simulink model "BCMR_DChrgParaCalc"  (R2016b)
settings: Solver=FixedStepDiscrete  StartTime=0.0  StopTime=10  FixedStep=0.01  RelTol=1e-3  EnableMultiTasking=on
undefined symbols (not defined in the file or in its folder): BCMR_ahDChgBattNominalCapa_C, BCMR_bCurrCalSelect_C, BCMR_bCurrIncDeltaLimEna_C, BCMR_bDChrgFulChkTenEna_C, BCMR_bDChrgFulChkThreeEna_C, BCMR_cntCoolDFC_CW, BCMR_cntSoh_CW, BCMR_G1E0PlatformSwPara_C, BCMR_iCurrDcr_C, BCMR_iDcChrgCurrAbnorm_T, BCMR_iDcChrgCurrAbnormMAP_T, BCMR_iDcChrgCurrNew_T, BCMR_iDcChrgCurrNewMAP_T, BCMR_iDcChrgCurrOld_T, BCMR_iDcChrgCurrOldAbnorm_T, BCMR_iDcChrgCurrOldAbnormMAP_T, BCMR_iDcChrgCurrOldMAP_T, BCMR_iDCCurrDecStep_C, BCMR_iDCCurrDecThrd_C, BCMR_iDCCurrDeltaLim_C, BCMR_iDCCurrDiff_C, BCMR_iDCCurrFil_C, BCMR_iDCCurrIncStep_C, BCMR_iDCCurrIncThrd_C, BCMR_iDChrgCurrCutOff_C, BCMR_kmAcmDist_C, BCMR_numCcsPwrSelc_C, BCMR_numCellVoltFull_C, BCMR_numCellVoltFullThree_C, BCMR_numCurrCalcEna, BCMR_pCcsPwrSelc_C, BCMR_pctBmsPwrRdc_C, BCMR_rCurrDcr_C, BCMR_rCurrIcr_C, BCMR_rDchrgLoadCoef_C, BCMR_tBattTempMaxFil_C, BCMR_tBattTempSelcLmtDwn_C, BCMR_tBattTempSelcLmtUp_C, BCMR_tDcChrgCellTemp1_A, BCMR_tDcChrgCellTemp2_A, BCMR_tDcChrgCellTemp_A, BCMR_tDchrgLoadLmt_C, BCMR_tiBattTempMaxFilDly_C, BCMR_tiBattTempSwitch_C, BCMR_tiCellVoltFullCnt_C, BCMR_tiCellVoltMaxFilDly_C, BCMR_tiCurrHysTimeDelay_C, BCMR_tiDcChrgPwrCCSDebs_C, BCMR_tiDChgFullPreHold_C, BCMR_tiDChrgCurrReqCalDly_C, BCMR_tiDChrgDetParaDebs_C, BCMR_tiDChrgFullBase_C, BCMR_tiDChrgFullDebs_C, BCMR_tiDChrgFulParaDebs_C, BCMR_tiDChrgFulWait_C, BCMR_tiDChrgParaBase_C, BCMR_tiHoldOnToCurrCalcOff_C, BCMR_tTempDisMapX_A, BCMR_tTempDisMapY_A, BCMR_uBattVoltOff_C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
libraries: simulink x34
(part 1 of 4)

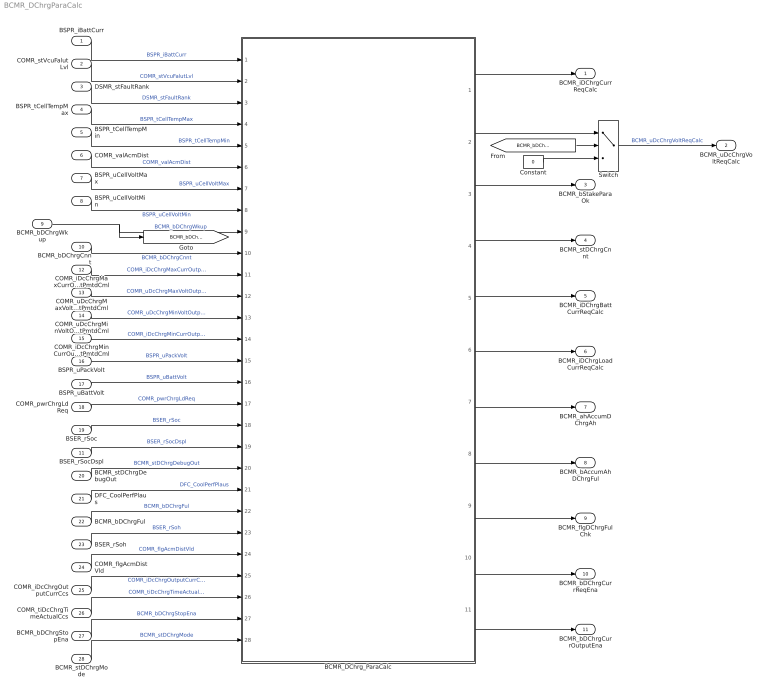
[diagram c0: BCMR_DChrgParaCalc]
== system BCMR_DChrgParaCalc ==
  BSPR_iBattCurr : Inport
  COMR_stVcuFalutLvl : Inport  Port=2
  DSMR_stFaultRank : Inport  Port=3
  BSPR_tCellTempMax : Inport  Port=4
  BSPR_tCellTempMin : Inport  Port=5
  COMR_valAcmDist : Inport  Port=6
  BSPR_uCellVoltMax : Inport  Port=7
  BSPR_uCellVoltMin : Inport  Port=8
  BCMR_bDChrgWkup : Inport  Port=9
  BCMR_bDChrgCnnt : Inport  Port=10
  BSER_rSocDspl : Inport  Port=11
  COMR_iDcChrgMaxCurrOutputPmtdCml : Inport  Port=12
  COMR_uDcChrgMaxVoltOutputPmtdCml : Inport  Port=13
  COMR_uDcChrgMinVoltOutputPmtdCml : Inport  Port=14
  COMR_iDcChrgMinCurrOutputPmtdCml : Inport  Port=15
  BSPR_uPackVolt : Inport  Port=16
  BSPR_uBattVolt : Inport  Port=17
  COMR_pwrChrgLdReq : Inport  Port=18
  BSER_rSoc : Inport  Port=19
  BCMR_stDChrgDebugOut : Inport  Port=20
  DFC_CoolPerfPlaus : Inport  Port=21
  BCMR_bDChrgFul : Inport  Port=22
  BSER_rSoh : Inport  Port=23
  COMR_flgAcmDistVld : Inport  Port=24
  COMR_iDcChrgOutputCurrCcs : Inport  Port=25
  COMR_tiDcChrgTimeActualCcs : Inport  Port=26
  BCMR_bDChrgStopEna : Inport  Port=27
  BCMR_stDChrgMode : Inport  Port=28
  BCMR_DChrg_ParaCalc : Subsystem
  Constant : Constant  Value=0
  Switch : Switch  Criteria=u2 > Threshold  OutDataTypeStr=single
  BCMR_iDChrgCurrReqCalc : Outport
  BCMR_uDcChrgVoltReqCalc : Outport  Port=2
  BCMR_bStakeParaOk : Outport  Port=3
  BCMR_stDChrgCnnt : Outport  Port=4
  BCMR_iDChrgBattCurrReqCalc : Outport  Port=5
  BCMR_iDChrgLoadCurrReqCalc : Outport  Port=6
  BCMR_ahAccumDChrgAh : Outport  Port=7  InitialOutput=[0]
  BCMR_bAccumAhDChrgFul : Outport  Port=8  InitialOutput=[0]
  BCMR_flgDChrgFulChk : Outport  Port=9
  BCMR_bDChrgCurrReqEna : Outport  Port=10  OutputWhenDisabled=reset  InitialOutput=[0]
  BCMR_bDChrgCurrOutputEna : Outport  Port=11  OutputWhenDisabled=reset  InitialOutput=[0]
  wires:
  BSPR_iBattCurr/1 -> BCMR_DChrg_ParaCalc/1(BSPR_iBattCurr)  "BSPR_iBattCurr"
  COMR_stVcuFalutLvl/1 -> BCMR_DChrg_ParaCalc/2(COMR_stVcuFalutLvl)  "COMR_stVcuFalutLvl"
  DSMR_stFaultRank/1 -> BCMR_DChrg_ParaCalc/3(DSMR_stFaultRank)  "DSMR_stFaultRank"
  BSPR_tCellTempMax/1 -> BCMR_DChrg_ParaCalc/4(BSPR_tBattTempMax)  "BSPR_tCellTempMax"
  BSPR_tCellTempMin/1 -> BCMR_DChrg_ParaCalc/5(BSPR_tBattTempMin)  "BSPR_tCellTempMin"
  COMR_valAcmDist/1 -> BCMR_DChrg_ParaCalc/6(COMR_valAcmDist)  "COMR_valAcmDist"
  BSPR_uCellVoltMax/1 -> BCMR_DChrg_ParaCalc/7(BSPR_uCellVoltMax)  "BSPR_uCellVoltMax"
  BSPR_uCellVoltMin/1 -> BCMR_DChrg_ParaCalc/8(BSPR_uCellVoltMin)  "BSPR_uCellVoltMin"
  BCMR_bDChrgWkup/1 -> [BCMR_bDChrgWkup], BCMR_DChrg_ParaCalc/9(BCMR_bDChrgWkup)  "BCMR_bDChrgWkup"
  BCMR_bDChrgCnnt/1 -> BCMR_DChrg_ParaCalc/10(BCMR_bDChrgCnnt)  "BCMR_bDChrgCnnt"
  BSER_rSocDspl/1 -> BCMR_DChrg_ParaCalc/19(BSER_rSocDspl)  "BSER_rSocDspl"
  COMR_iDcChrgMaxCurrOutputPmtdCml/1 -> BCMR_DChrg_ParaCalc/11(COMR_iDcChrgMaxCurrOutputPmtdCml)  "COMR_iDcChrgMaxCurrOutputPmtdCml"
  COMR_uDcChrgMaxVoltOutputPmtdCml/1 -> BCMR_DChrg_ParaCalc/12(COMR_uDcChrgMaxVoltOutputPmtdCml)  "COMR_uDcChrgMaxVoltOutputPmtdCml"
  COMR_uDcChrgMinVoltOutputPmtdCml/1 -> BCMR_DChrg_ParaCalc/13(COMR_uDcChrgMinVoltOutputPmtdCml)  "COMR_uDcChrgMinVoltOutputPmtdCml"
  COMR_iDcChrgMinCurrOutputPmtdCml/1 -> BCMR_DChrg_ParaCalc/14(COMR_iDcChrgMinCurrOutputPmtdCml)  "COMR_iDcChrgMinCurrOutputPmtdCml"
  BSPR_uPackVolt/1 -> BCMR_DChrg_ParaCalc/15(BSPR_uPackVolt)  "BSPR_uPackVolt"
  BSPR_uBattVolt/1 -> BCMR_DChrg_ParaCalc/16(BSPR_uBattVolt)  "BSPR_uBattVolt"
  BCMR_DChrg_ParaCalc/1(BCMR_iDChrgCurrReqCalc) -> BCMR_iDChrgCurrReqCalc/1
  BCMR_DChrg_ParaCalc/3(BCMR_bStakeParaOk) -> BCMR_bStakeParaOk/1
  BCMR_DChrg_ParaCalc/4("BCMR_stDChrgCnnt ") -> BCMR_stDChrgCnnt/1
  COMR_pwrChrgLdReq/1 -> BCMR_DChrg_ParaCalc/17(COMR_pwrChrgLdReq)  "COMR_pwrChrgLdReq"
  BCMR_DChrg_ParaCalc/5(BCMR_iDChrgBattCurrReqCalc) -> BCMR_iDChrgBattCurrReqCalc/1
  BCMR_DChrg_ParaCalc/6(BCMR_iDChrgLoadCurrReqCalc) -> BCMR_iDChrgLoadCurrReqCalc/1
  BSER_rSoc/1 -> BCMR_DChrg_ParaCalc/18(BSER_rSoc)  "BSER_rSoc"
  BCMR_DChrg_ParaCalc/7(BCMR_ahAccumDChrgAh) -> BCMR_ahAccumDChrgAh/1
  BCMR_DChrg_ParaCalc/8(BCMR_bAccumAhDChrgFul) -> BCMR_bAccumAhDChrgFul/1
  BCMR_DChrg_ParaCalc/9(BCMR_flgDChrgFulChk) -> BCMR_flgDChrgFulChk/1
  BCMR_stDChrgDebugOut/1 -> BCMR_DChrg_ParaCalc/20(BCMR_stDChrgDebugOut)  "BCMR_stDChrgDebugOut"
  DFC_CoolPerfPlaus/1 -> BCMR_DChrg_ParaCalc/21(DFC_CoolPerfPlaus)  "DFC_CoolPerfPlaus"
  BCMR_bDChrgFul/1 -> BCMR_DChrg_ParaCalc/22(BCMR_bDChrgFul)  "BCMR_bDChrgFul"
  BSER_rSoh/1 -> BCMR_DChrg_ParaCalc/23(BSER_rSoh)  "BSER_rSoh"
  BCMR_DChrg_ParaCalc/10(BCMR_bDChrgCurrReqEna) -> BCMR_bDChrgCurrReqEna/1
  BCMR_DChrg_ParaCalc/11(BCMR_bDChrgCurrOutputEna) -> BCMR_bDChrgCurrOutputEna/1
  COMR_flgAcmDistVld/1 -> BCMR_DChrg_ParaCalc/24(COMR_flgAcmDistVld)  "COMR_flgAcmDistVld"
  COMR_iDcChrgOutputCurrCcs/1 -> BCMR_DChrg_ParaCalc/25(COMR_iDcChrgOutputCurrCcs)  "COMR_iDcChrgOutputCurrCcs"
  COMR_tiDcChrgTimeActualCcs/1 -> BCMR_DChrg_ParaCalc/26(COMR_tiDcChrgTimeActualCcs)  "COMR_tiDcChrgTimeActualCcs"
  BCMR_bDChrgStopEna/1 -> BCMR_DChrg_ParaCalc/27(BCMR_bDChrgStopEna)  "BCMR_bDChrgStopEna"
  BCMR_stDChrgMode/1 -> BCMR_DChrg_ParaCalc/28(BCMR_stDChrgMode)  "BCMR_stDChrgMode"
  Switch/1 -> BCMR_uDcChrgVoltReqCalc/1  "BCMR_uDcChrgVoltReqCalc"
  [BCMR_bDChrgWkup] -> Switch/2
  Constant/1 -> Switch/3
  BCMR_DChrg_ParaCalc/2(BCMR_uDcChrgVoltReqCalc) -> Switch/1

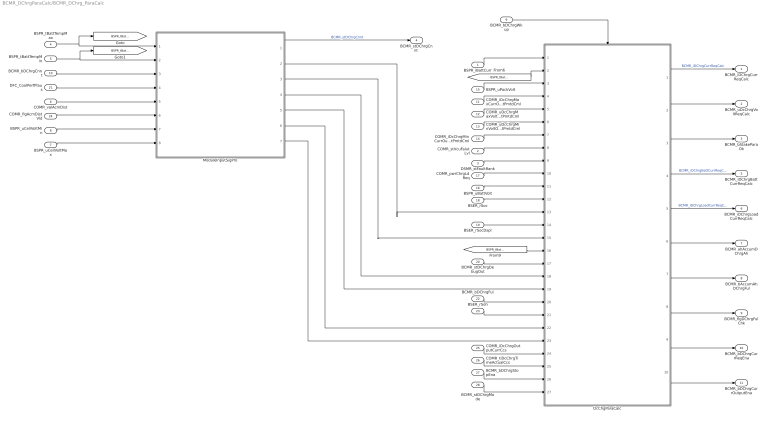
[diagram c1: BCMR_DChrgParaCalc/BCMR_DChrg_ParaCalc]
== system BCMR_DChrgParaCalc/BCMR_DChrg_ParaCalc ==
  BSPR_iBattCurr : Inport
  COMR_stVcuFalutLvl : Inport  Port=2
  DSMR_stFaultRank : Inport  Port=3
  BSPR_tBattTempMax : Inport  Port=4
  BSPR_tBattTempMin : Inport  Port=5
  COMR_valAcmDist : Inport  Port=6
  BSPR_uCellVoltMax : Inport  Port=7
  BSPR_uCellVoltMin : Inport  Port=8
  BCMR_bDChrgWkup : Inport  Port=9
  BCMR_bDChrgCnnt : Inport  Port=10
  COMR_iDcChrgMaxCurrOutputPmtdCml : Inport  Port=11
  COMR_uDcChrgMaxVoltOutputPmtdCml : Inport  Port=12
  COMR_uDcChrgMinVoltOutputPmtdCml : Inport  Port=13
  COMR_iDcChrgMinCurrOutputPmtdCml : Inport  Port=14
  BSPR_uPackVolt : Inport  Port=15
  BSPR_uBattVolt : Inport  Port=16
  COMR_pwrChrgLdReq : Inport  Port=17
  BSER_rSoc : Inport  Port=18
  BSER_rSocDspl : Inport  Port=19
  BCMR_stDChrgDebugOut : Inport  Port=20
  DFC_CoolPerfPlaus : Inport  Port=21
  BCMR_bDChrgFul : Inport  Port=22
  BSER_rSoh : Inport  Port=23
  COMR_flgAcmDistVld : Inport  Port=24
  COMR_iDcChrgOutputCurrCcs : Inport  Port=25
  COMR_tiDcChrgTimeActualCcs : Inport  Port=26
  BCMR_bDChrgStopEna : Inport  Port=27
  BCMR_stDChrgMode : Inport  Port=28
  DcChgParaCalc : Subsystem  TreatAsAtomicUnit=on
  ModuleInputSigPro : Subsystem  TreatAsAtomicUnit=on
  BCMR_iDChrgCurrReqCalc : Outport
  BCMR_uDcChrgVoltReqCalc : Outport  Port=2
  BCMR_bStakeParaOk : Outport  Port=3
  "BCMR_stDChrgCnnt " : Outport  Port=4
  BCMR_iDChrgBattCurrReqCalc : Outport  Port=5
  BCMR_iDChrgLoadCurrReqCalc : Outport  Port=6
  BCMR_ahAccumDChrgAh : Outport  Port=7  InitialOutput=[0]
  BCMR_bAccumAhDChrgFul : Outport  Port=8  InitialOutput=[0]
  BCMR_flgDChrgFulChk : Outport  Port=9
  BCMR_bDChrgCurrReqEna : Outport  Port=10  OutputWhenDisabled=reset  InitialOutput=[0]
  BCMR_bDChrgCurrOutputEna : Outport  Port=11  OutputWhenDisabled=reset  InitialOutput=[0]
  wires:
  BCMR_bDChrgWkup/1 -> DcChgParaCalc/Enable
  ModuleInputSigPro/1(BCMR_stDChrgCnnt) -> "BCMR_stDChrgCnnt "/1  "BCMR_stDChrgCnnt"
  BSPR_iBattCurr/1 -> DcChgParaCalc/1(BSPR_iBattCurr)
  BSPR_uBattVolt/1 -> DcChgParaCalc/11(BSPR_uBattVolt)
  BSPR_uPackVolt/1 -> DcChgParaCalc/3(BSPR_uPackVolt)
  COMR_iDcChrgMaxCurrOutputPmtdCml/1 -> DcChgParaCalc/4(COMR_iDcChrgMaxCurrOutputPmtdCml)
  COMR_uDcChrgMaxVoltOutputPmtdCml/1 -> DcChgParaCalc/5(COMR_uDcChrgMaxVoltOutputPmtdCml)
  COMR_uDcChrgMinVoltOutputPmtdCml/1 -> DcChgParaCalc/6(COMR_uDcChrgMinVoltOutputPmtdCml)
  COMR_iDcChrgMinCurrOutputPmtdCml/1 -> DcChgParaCalc/7(COMR_iDcChrgMinCurrOutputPmtdCml)
  COMR_stVcuFalutLvl/1 -> DcChgParaCalc/8(COMR_stVcuFalutLvl)
  DSMR_stFaultRank/1 -> DcChgParaCalc/9(DSMR_stFaultRank)
  DcChgParaCalc/2(BCMR_uDcChrgVoltReqCalc) -> BCMR_uDcChrgVoltReqCalc/1
  DcChgParaCalc/1(BCMR_iDChrgCurrReqCalc) -> BCMR_iDChrgCurrReqCalc/1  "BCMR_iDChrgCurrReqCalc"
  DcChgParaCalc/3(BCMR_bStakeParaOk) -> BCMR_bStakeParaOk/1
  COMR_pwrChrgLdReq/1 -> DcChgParaCalc/10(COMR_pwrChrgLdReq)
  DcChgParaCalc/4(BCMR_iDChrgBattCurrReqCalc) -> BCMR_iDChrgBattCurrReqCalc/1  "BCMR_iDChrgBattCurrReqCalc"
  DcChgParaCalc/5(BCMR_iDChrgLoadCurrReqCalc) -> BCMR_iDChrgLoadCurrReqCalc/1  "BCMR_iDChrgLoadCurrReqCalc"
  BSER_rSoc/1 -> DcChgParaCalc/12(BSER_rSoc)
  DcChgParaCalc/6(BCMR_ahAccumDChrgAh) -> BCMR_ahAccumDChrgAh/1
  DcChgParaCalc/7(BCMR_bAccumAhDChrgFul) -> BCMR_bAccumAhDChrgFul/1
  DcChgParaCalc/8(BCMR_flgDChrgFulChk) -> BCMR_flgDChrgFulChk/1
  BSER_rSocDspl/1 -> DcChgParaCalc/14(BSER_rSocDspl)
  BSPR_tBattTempMax/1 -> [BSPR_tBattTempMax], ModuleInputSigPro/1(BSPR_tBattTempMax)
  BSPR_tBattTempMin/1 -> ModuleInputSigPro/2(BSPR_tBattTempMin), [BSPR_tBattTempMin]
  [BSPR_tBattTempMin] -> DcChgParaCalc/2(BSPR_tBattTempMin)
  BSPR_uCellVoltMax/1 -> ModuleInputSigPro/8(BSPR_uCellVoltMin)
  [BSPR_tBattTempMax] -> DcChgParaCalc/16(BSPR_tBattTempMax)
  BSPR_uCellVoltMin/1 -> ModuleInputSigPro/7(BSPR_uCellVoltMax)
  BCMR_stDChrgDebugOut/1 -> DcChgParaCalc/17(BCMR_stDChrgDebugOut)
  ModuleInputSigPro/4(BCMR_uDcChrgCellVolt_A) -> DcChgParaCalc/18(BCMR_uDcChrgCellVolt_A)
  DFC_CoolPerfPlaus/1 -> ModuleInputSigPro/4(DFC_CoolPerfPlaus)
  ModuleInputSigPro/5(BCMR_bDChrgCoolAbnorm) -> DcChgParaCalc/19(BCMR_bDChrgCoolAbnorm)
  BCMR_bDChrgFul/1 -> DcChgParaCalc/20(BCMR_bDChrgFul)
  BSER_rSoh/1 -> DcChgParaCalc/21(BSER_rSoh)
  DcChgParaCalc/9(BCMR_bDChrgCurrReqEna) -> BCMR_bDChrgCurrReqEna/1
  DcChgParaCalc/10(BCMR_bDChrgCurrOutputEna) -> BCMR_bDChrgCurrOutputEna/1
  BCMR_bDChrgCnnt/1 -> ModuleInputSigPro/3(BCMR_bDChrgCnnt)
  COMR_valAcmDist/1 -> ModuleInputSigPro/5(COMR_valAcmDist)
  COMR_flgAcmDistVld/1 -> ModuleInputSigPro/6(COMR_flgAcmDistVld)
  ModuleInputSigPro/6(BCMR_tDcChrgCellTemp_A) -> DcChgParaCalc/22(BCMR_tDcChrgCellTemp_A)
  ModuleInputSigPro/7(BCMR_bDChrgDistLmt) -> DcChgParaCalc/23(BCMR_bDChrgDistLmt)
  COMR_tiDcChrgTimeActualCcs/1 -> DcChgParaCalc/25(COMR_tiDcChrgTimeActualCcs)
  COMR_iDcChrgOutputCurrCcs/1 -> DcChgParaCalc/24(COMR_iDcChrgOutputCurrCcs)
  BCMR_bDChrgStopEna/1 -> DcChgParaCalc/26(BCMR_bDChrgStopEna)
  BCMR_stDChrgMode/1 -> DcChgParaCalc/27(BCMR_stDChrgMode)
  ModuleInputSigPro/2(BCMR_uCellVoltMax) -> DcChgParaCalc/13(BSPR_uCellVoltMax)
  ModuleInputSigPro/3(BCMR_uCellVoltMin) -> DcChgParaCalc/15(BSPR_uCellVoltMin)

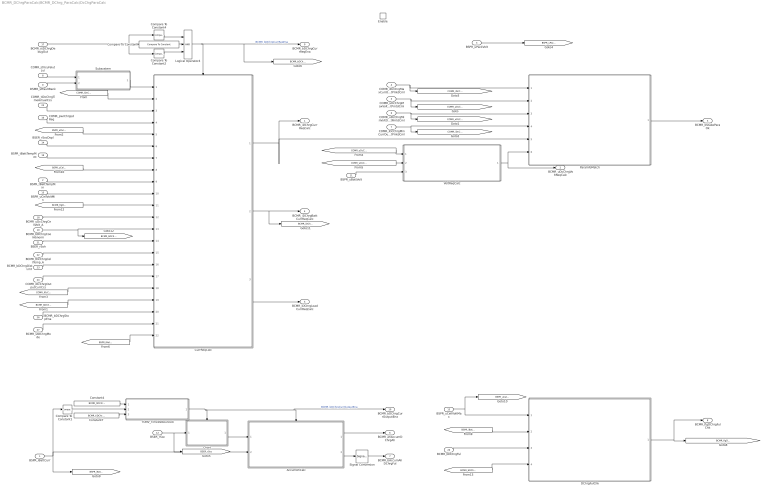
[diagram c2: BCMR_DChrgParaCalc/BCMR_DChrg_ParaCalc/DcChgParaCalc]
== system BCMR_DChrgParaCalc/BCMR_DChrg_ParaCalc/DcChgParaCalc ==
  BSPR_iBattCurr : Inport
  BSPR_tBattTempMin : Inport  Port=2
  BSPR_uPackVolt : Inport  Port=3
  COMR_iDcChrgMaxCurrOutputPmtdCml : Inport  Port=4
  COMR_uDcChrgMaxVoltOutputPmtdCml : Inport  Port=5
  COMR_uDcChrgMinVoltOutputPmtdCml : Inport  Port=6
  COMR_iDcChrgMinCurrOutputPmtdCml : Inport  Port=7
  COMR_stVcuFalutLvl : Inport  Port=8
  DSMR_stFaultRank : Inport  Port=9
  COMR_pwrChrgLdReq : Inport  Port=10
  BSPR_uBattVolt : Inport  Port=11
  BSER_rSoc : Inport  Port=12
  BSPR_uCellVoltMax : Inport  Port=13
  BSER_rSocDspl : Inport  Port=14
  BSPR_uCellVoltMin : Inport  Port=15
  BSPR_tBattTempMax : Inport  Port=16
  BCMR_stDChrgDebugOut : Inport  Port=17
  BCMR_uDcChrgCellVolt_A : Inport  Port=18
  BCMR_bDChrgCoolAbnorm : Inport  Port=19
  BCMR_bDChrgFul : Inport  Port=20
  BSER_rSoh : Inport  Port=21
  BCMR_tDcChrgCellTemp_A : Inport  Port=22
  BCMR_bDChrgDistLmt : Inport  Port=23
  COMR_iDcChrgOutputCurrCcs : Inport  Port=24
  COMR_tiDcChrgTimeActualCcs : Inport  Port=25
  BCMR_bDChrgStopEna : Inport  Port=26
  BCMR_stDChrgMode : Inport  Port=27
  Enable : EnablePort  StatesWhenEnabling=reset
  AccumAhCalc : Subsystem  TreatAsAtomicUnit=on
  Chart : Stateflow chart  TreatAsAtomicUnit=on
  Compare To Constant : simulink/Logic and Bit Operations/Compare To Constant  relop=>=  const=BCMR_numCurrCalcEna  OutDataTypeStr=boolean
  Compare To Constant1 : simulink/Logic and Bit Operations/Compare To Constant  relop=<=  const=-5  OutDataTypeStr=boolean
  Compare To Constant2 : simulink/Logic and Bit Operations/Compare To Constant  relop=<  const=34  OutDataTypeStr=boolean
  Compare To Constant4 : simulink/Logic and Bit Operations/Compare To Constant  relop=~=  const=24  OutDataTypeStr=boolean
  Constant4 : Constant  Value=BCMR_tiDChrgDetParaDebs_C
  Constant7 : Constant  Value=BCMR_tiDChrgParaBase_C
  CurrReqCalc : Subsystem  TreatAsAtomicUnit=on
  DChrgFulChk : Subsystem  TreatAsAtomicUnit=on
  Logical Operator4 : Logic  Inputs=3  AllPortsSameDT=off  OutDataTypeStr=boolean
  ParaInfoMatch : Subsystem
  Signal Conversion : SignalConversion  OverrideOpt=off
  Subsystem : Subsystem
  TONV_TimeDebounce4 : Subsystem  TreatAsAtomicUnit=on
  VoltReqCalc : Subsystem  TreatAsAtomicUnit=on
  BCMR_iDChrgCurrReqCalc : Outport  OutputWhenDisabled=reset  InitialOutput=[0]
  BCMR_uDcChrgVoltReqCalc : Outport  Port=2  InitialOutput=[0]
  BCMR_bStakeParaOk : Outport  Port=3  OutputWhenDisabled=reset  InitialOutput=[0]
  BCMR_iDChrgBattCurrReqCalc : Outport  Port=4  OutputWhenDisabled=reset  InitialOutput=[0]
  BCMR_iDChrgLoadCurrReqCalc : Outport  Port=5  OutputWhenDisabled=reset  InitialOutput=[0]
  BCMR_ahAccumDChrgAh : Outport  Port=6  OutputWhenDisabled=reset  InitialOutput=[0]
  BCMR_bAccumAhDChrgFul : Outport  Port=7  InitialOutput=[0]
  BCMR_flgDChrgFulChk : Outport  Port=8  OutputWhenDisabled=reset  InitialOutput=[0]
  BCMR_bDChrgCurrReqEna : Outport  Port=9  OutputWhenDisabled=reset  InitialOutput=[0]
  BCMR_bDChrgCurrOutputEna : Outport  Port=10  OutputWhenDisabled=reset  InitialOutput=[0]
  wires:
  VoltReqCalc/1(BCMR_uDcChrgVoltReqCalc) -> ParaInfoMatch/6(BCMR_uDcChrgVoltReqCalc), BCMR_uDcChrgVoltReqCalc/1
  ParaInfoMatch/1(BCMR_bStakeParaOk) -> BCMR_bStakeParaOk/1
  COMR_uDcChrgMaxVoltOutputPmtdCml/1 -> [COMR_uDcChrgMaxVoltOutputPmtdCml], ParaInfoMatch/2(COMR_uDcChrgMaxVoltOutputPmtdCml)
  COMR_uDcChrgMinVoltOutputPmtdCml/1 -> [COMR_uDcChrgMinVoltOutputPmtdCml], ParaInfoMatch/3(COMR_uDcChrgMinVoltOutputPmtdCml)
  [COMR_uDcChrgMaxVoltOutputPmtdCml] -> VoltReqCalc/1(COMR_uDcChrgMaxVoltOutputPmtdCml)
  [COMR_uDcChrgMinVoltOutputPmtdCml] -> VoltReqCalc/2(COMR_uDcChrgMinVoltOutputPmtdCml)
  COMR_iDcChrgMaxCurrOutputPmtdCml/1 -> ParaInfoMatch/1(COMR_iDcChrgMaxCurrOutputPmtdCml), [COMR_iDcChrgMaxCurrOutputPmtdCml]
  COMR_iDcChrgMinCurrOutputPmtdCml/1 -> [COMR_iDcChrgMinCurrOutputPmtdCml], ParaInfoMatch/4(COMR_iDcChrgMinCurrOutputPmtdCml)
  BSPR_uPackVolt/1 -> [BSPR_uPackVolt]
  BSPR_iBattCurr/1 -> AccumAhCalc/2(BSPR_iBattCurr), [BSPR_iBattCurr], Compare To Constant1/1
  [COMR_iDcChrgMaxCurrOutputPmtdCml] -> CurrReqCalc/2(COMR_iDcChrgMaxCurrOutputPmtdCml)
  COMR_stVcuFalutLvl/1 -> Subsystem/1(COMR_stVcuFalutLvl)
  DSMR_stFaultRank/1 -> Subsystem/2(DSMR_stFaultRank)
  Subsystem/1(BCMR_flgDChrgPwrRdc) -> CurrReqCalc/1(BCMR_flgDChrgPwrRdc)
  [BSPR_uPackVolt] -> CurrReqCalc/5(BSPR_uPackVolt)
  COMR_pwrChrgLdReq/1 -> CurrReqCalc/4(COMR_pwrChrgLdReq)
  CurrReqCalc/3(BCMR_iDChrgLoadCurrReqCalc) -> BCMR_iDChrgLoadCurrReqCalc/1
  CurrReqCalc/2(BCMR_iDChrgBattCurrReqCalc) -> BCMR_iDChrgBattCurrReqCalc/1, [BCMR_iDChrgBattCurrReqCalc]
  BSER_rSoc/1 -> [BSER_rSoc], Chart/1(BSER_rSoc)
  Chart/1(BCMR_rSocInit) -> AccumAhCalc/1(BCMR_rSocInit)
  AccumAhCalc/1(BCMR_ahAccumDChrgAh) -> BCMR_ahAccumDChrgAh/1
  AccumAhCalc/2(BCMR_bAccumAhDChrgFul) -> Signal Conversion/1
  BSER_rSocDspl/1 -> CurrReqCalc/6(BSER_rSocDspl)
  Compare To Constant1/1 -> TONV_TimeDebounce4/2(u)
  TONV_TimeDebounce4/1(y) -> BCMR_bDChrgCurrOutputEna/1, AccumAhCalc/Enable, Chart/Trigger  "BCMR_bDChrgCurrOutputEna"
  Constant7/1 -> TONV_TimeDebounce4/3(dT)
  Constant4/1 -> TONV_TimeDebounce4/1(T)
  BSPR_tBattTempMin/1 -> CurrReqCalc/9(BSPR_tBattTempMin)
  BSPR_uCellVoltMin/1 -> CurrReqCalc/10(BSPR_uCellVoltMin)
  [BSPR_uCellVoltMax] -> CurrReqCalc/8(BSPR_uCellVoltMax)
  BSPR_tBattTempMax/1 -> CurrReqCalc/7(BSPR_tBattTempMax)
  [BCMR_flgDChrgFulChk] -> CurrReqCalc/11(BCMR_flgDChrgFulChk)
  DChrgFulChk/1(BCMR_flgDChrgFulChk) -> BCMR_flgDChrgFulChk/1, [BCMR_flgDChrgFulChk]
  BCMR_stDChrgDebugOut/1 -> Compare To Constant4/1, Compare To Constant/1, Compare To Constant2/1
  COMR_tiDcChrgTimeActualCcs/1 -> CurrReqCalc/3(COMR_tiDcChrgTimeActualCcs)
  BCMR_uDcChrgCellVolt_A/1 -> CurrReqCalc/12(BCMR_uDcChrgCellVolt_A)
  [BSPR_iBattCurr] -> DChrgFulChk/2(BSPR_iBattCurr)
  BSPR_uCellVoltMax/1 -> DChrgFulChk/1(BSPR_uCellVoltMax), [BSPR_uCellVoltMax]
  BCMR_bDChrgFul/1 -> DChrgFulChk/3(BCMR_bDChrgFul)
  BSER_rSoh/1 -> CurrReqCalc/14(BSER_rSoh)
  [BCMR_bDChrgCoolAbnorm] -> DChrgFulChk/4(BCMR_bDChrgCoolAbnorm)
  Logical Operator4/1 -> [BCMR_bDChrgCurrReqEna], BCMR_bDChrgCurrReqEna/1, CurrReqCalc/Enable  "BCMR_bDChrgCurrReqEna"
  Compare To Constant4/1 -> Logical Operator4/1
  Compare To Constant/1 -> Logical Operator4/2
  Compare To Constant2/1 -> Logical Operator4/3
  BCMR_bDChrgCoolAbnorm/1 -> [BCMR_bDChrgCoolAbnorm], CurrReqCalc/13(BCMR_bDChrgCoolAbnorm)
  CurrReqCalc/1(BCMR_iDChrgCurrReqCalc) -> ParaInfoMatch/5(BCMR_iDChrgCurrReqCalc), BCMR_iDChrgCurrReqCalc/1
  BCMR_tDcChrgCellTemp_A/1 -> CurrReqCalc/15(BCMR_tDcChrgCellTemp_A)
  BCMR_bDChrgDistLmt/1 -> CurrReqCalc/16(BCMR_bDChrgDistLmt)
  BSPR_uBattVolt/1 -> VoltReqCalc/3(BSPR_uBattVolt)
  [COMR_iDcChrgMinCurrOutputPmtdCml] -> CurrReqCalc/18(COMR_iDcChrgMinCurrOutputPmtdCml)
  COMR_iDcChrgOutputCurrCcs/1 -> CurrReqCalc/17(COMR_iDcChrgOutputCurrCcs)
  [BCMR_bDChrgCurrReqEna] -> CurrReqCalc/19(BCMR_bDChrgCurrReqEna)
  BCMR_bDChrgStopEna/1 -> CurrReqCalc/20(BCMR_bDChrgStopEna)
  BCMR_stDChrgMode/1 -> CurrReqCalc/21(BCMR_stDChrgMode)
  [BSPR_iBattCurr] -> CurrReqCalc/22(BSPR_iBattCurr)
  Signal Conversion/1 -> BCMR_bAccumAhDChrgFul/1

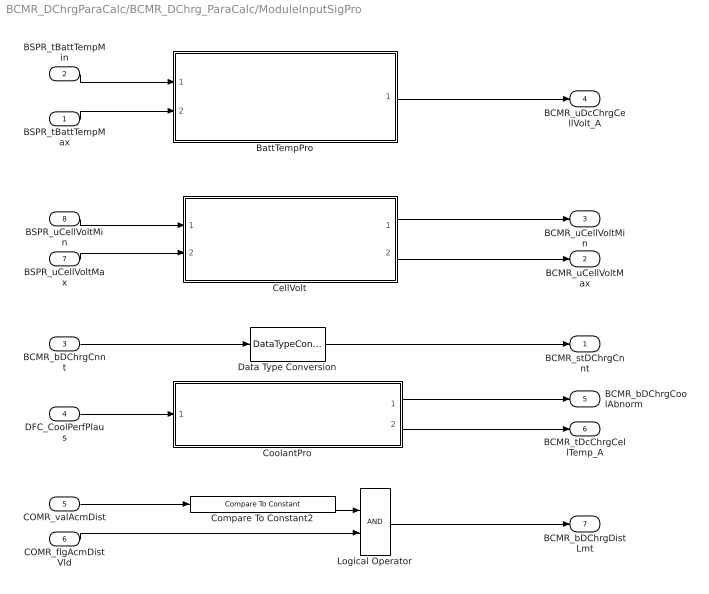
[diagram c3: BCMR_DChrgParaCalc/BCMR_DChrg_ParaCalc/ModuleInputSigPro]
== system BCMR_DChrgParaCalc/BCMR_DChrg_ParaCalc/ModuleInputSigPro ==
  BSPR_tBattTempMax : Inport
  BSPR_tBattTempMin : Inport  Port=2
  BCMR_bDChrgCnnt : Inport  Port=3
  DFC_CoolPerfPlaus : Inport  Port=4
  COMR_valAcmDist : Inport  Port=5
  COMR_flgAcmDistVld : Inport  Port=6
  BSPR_uCellVoltMax : Inport  Port=7
  BSPR_uCellVoltMin : Inport  Port=8
  BattTempPro : Subsystem
  CellVolt : Subsystem
  Compare To Constant2 : simulink/Logic and Bit Operations/Compare To Constant  relop=>=  const=BCMR_kmAcmDist_C  OutDataTypeStr=boolean
  CoolantPro : Subsystem
  Data Type Conversion : DataTypeConversion  OutDataTypeStr=uint8
  Logical Operator : Logic  AllPortsSameDT=off  OutDataTypeStr=boolean
  BCMR_stDChrgCnnt : Outport
  BCMR_uCellVoltMax : Outport  Port=2
  BCMR_uCellVoltMin : Outport  Port=3
  BCMR_uDcChrgCellVolt_A : Outport  Port=4
  BCMR_bDChrgCoolAbnorm : Outport  Port=5
  BCMR_tDcChrgCellTemp_A : Outport  Port=6
  BCMR_bDChrgDistLmt : Outport  Port=7
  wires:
  BSPR_tBattTempMin/1 -> BattTempPro/1(BSPR_tBattTempMin)
  BCMR_bDChrgCnnt/1 -> Data Type Conversion/1
  Data Type Conversion/1 -> BCMR_stDChrgCnnt/1
  BSPR_tBattTempMax/1 -> BattTempPro/2(BSPR_tBattTempMax)
  BattTempPro/1(BCMR_uDcChrgCellVolt_A) -> BCMR_uDcChrgCellVolt_A/1
  DFC_CoolPerfPlaus/1 -> CoolantPro/1(DFC_CoolPerfPlaus)
  CoolantPro/1(BCMR_bDChrgCoolAbnorm) -> BCMR_bDChrgCoolAbnorm/1
  CoolantPro/2(BCMR_uDcChrgCellTemp_A) -> BCMR_tDcChrgCellTemp_A/1
  COMR_valAcmDist/1 -> Compare To Constant2/1
  COMR_flgAcmDistVld/1 -> Logical Operator/2
  Compare To Constant2/1 -> Logical Operator/1
  Logical Operator/1 -> BCMR_bDChrgDistLmt/1
  BSPR_uCellVoltMax/1 -> CellVolt/2(BSPR_uCellVoltMin)
  BSPR_uCellVoltMin/1 -> CellVolt/1(BSPR_uCellVoltMax)
  CellVolt/1(BCMR_uCellVoltMin) -> BCMR_uCellVoltMin/1
  CellVolt/2(BCMR_uCellVoltMax) -> BCMR_uCellVoltMax/1

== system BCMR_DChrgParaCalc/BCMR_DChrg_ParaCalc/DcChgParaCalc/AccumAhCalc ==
  BCMR_rSocInit : Inport
  BSPR_iBattCurr : Inport  Port=2
  Enable : EnablePort  StatesWhenEnabling=reset
  AccmAh : Subsystem
  AccmAhChgFulChk : Subsystem
  BCMR_ahAccumDChrgAh : Outport
  BCMR_bAccumAhDChrgFul : Outport  Port=2  InitialOutput=[0]
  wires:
  AccmAh/1(BCMR_ahDChrgAhAccum) -> AccmAhChgFulChk/2(BCMR_ahAccumDChrgAh), BCMR_ahAccumDChrgAh/1  "BCMR_ahAccumDChrgAh"
  BSPR_iBattCurr/1 -> AccmAh/1(BSPR_iBattCurr)
  BCMR_rSocInit/1 -> AccmAhChgFulChk/1(BCMR_rSocInit)
  AccmAhChgFulChk/1(BCMR_bAccumAhDChrgFul) -> BCMR_bAccumAhDChrgFul/1

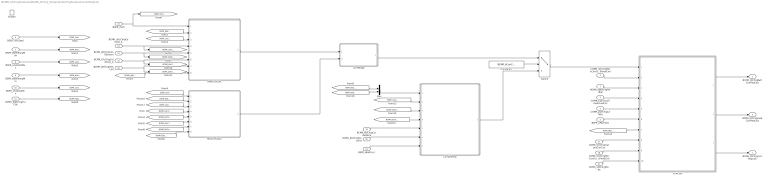
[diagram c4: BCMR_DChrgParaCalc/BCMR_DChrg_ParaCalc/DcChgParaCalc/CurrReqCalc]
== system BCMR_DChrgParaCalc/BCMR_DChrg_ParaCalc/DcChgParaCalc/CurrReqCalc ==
  BCMR_flgDChrgPwrRdc : Inport
  COMR_iDcChrgMaxCurrOutputPmtdCml : Inport  Port=2
  COMR_tiDcChrgTimeActualCcs : Inport  Port=3
  COMR_pwrChrgLdReq : Inport  Port=4
  BSPR_uPackVolt : Inport  Port=5
  BSER_rSocDspl : Inport  Port=6
  BSPR_tBattTempMax : Inport  Port=7
  BSPR_uCellVoltMax : Inport  Port=8
  BSPR_tBattTempMin : Inport  Port=9
  BSPR_uCellVoltMin : Inport  Port=10
  BCMR_flgDChrgFulChk : Inport  Port=11
  BCMR_uDcChrgCellVolt_A : Inport  Port=12
  BCMR_bDChrgCoolAbnorm : Inport  Port=13
  BSER_rSoh : Inport  Port=14
  BCMR_tDcChrgCellTemp_A : Inport  Port=15
  BCMR_bDChrgDistLmt : Inport  Port=16
  COMR_iDcChrgOutputCurrCcs : Inport  Port=17
  COMR_iDcChrgMinCurrOutputPmtdCml : Inport  Port=18
  BCMR_bDChrgCurrReqEna : Inport  Port=19
  BCMR_bDChrgStopEna : Inport  Port=20
  BCMR_stDChrgMode : Inport  Port=21
  BSPR_iBattCurr : Inport  Port=22
  Enable : EnablePort  StatesWhenEnabling=reset
  Constant1 : Constant  Value=BCMR_bCurrCalSelect_C
  CurrCalc : Subsystem
  CurrMerge : Subsystem
  CurrSpTemp : Subsystem
  MaxCurrCalc : Subsystem
  MixCurrCalc2 : Subsystem
  Mux : Mux  Inputs=2
  Switch : Switch  Criteria=u2 ~= 0
  BCMR_iDChrgCurrReqCalc : Outport  OutputWhenDisabled=reset  InitialOutput=[0]
  BCMR_iDChrgBattCurrReqCalc : Outport  Port=2  OutputWhenDisabled=reset  InitialOutput=[0]
  BCMR_iDChrgLoadCurrReqCalc : Outport  Port=3  OutputWhenDisabled=reset  InitialOutput=[0]
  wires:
  COMR_iDcChrgMaxCurrOutputPmtdCml/1 -> CurrCalc/2(COMR_iDcChrgMaxCurrOutputPmtdCml)
  BCMR_flgDChrgPwrRdc/1 -> CurrCalc/3(BCMR_flgDChrgPwrRdc)
  COMR_tiDcChrgTimeActualCcs/1 -> CurrCalc/4(COMR_tiDcChrgTimeActualCcs)
  COMR_pwrChrgLdReq/1 -> CurrCalc/5(COMR_pwrChrgLdReq)
  BSPR_uPackVolt/1 -> CurrCalc/6(BSPR_uPackVolt)
  CurrCalc/3(BCMR_iDChrgCurrReqCalc) -> BCMR_iDChrgCurrReqCalc/1
  CurrCalc/2(BCMR_iDChrgLoadCurrReqCalc) -> BCMR_iDChrgLoadCurrReqCalc/1
  CurrCalc/1(BCMR_iDChrgBattCurrReqCalc) -> BCMR_iDChrgBattCurrReqCalc/1
  BSER_rSocDspl/1 -> [BSER_rSocDspl]
  BSPR_uCellVoltMin/1 -> [BSPR_uCellVoltMin]
  BSPR_tBattTempMin/1 -> [BSPR_tBattTempMin]
  BSPR_uCellVoltMax/1 -> [BSPR_uCellVoltMax]
  BSPR_tBattTempMax/1 -> [BSPR_tBattTempMax]
  [BSPR_tBattTempMax] -> MaxCurrCalc/2(BSPR_tBattTempMax)
  [BSPR_uCellVoltMax] -> MaxCurrCalc/3(BSPR_uCellVoltMax)
  [BSPR_tBattTempMin] -> MixCurrCalc2/2(BSPR_tBattTempMax)
  [BSPR_uCellVoltMax] -> MixCurrCalc2/3(BSPR_uCellVoltMax)
  MixCurrCalc2/1(DChrgCurrCalcMix2) -> CurrMerge/2(In2)
  BCMR_flgDChrgFulChk/1 -> [BCMR_flgDChrgFulChk]
  [BSPR_tBattTempMin] -> CurrCalc/7(BSPR_tBattTempMin)
  MaxCurrCalc/1(DChrgCurrCalcMax) -> CurrMerge/1(In1)
  BCMR_uDcChrgCellVolt_A/1 -> [BCMR_uDcChrgCellVolt_A], MaxCurrCalc/4(BCMR_uDcChrgCellVolt_A)
  BCMR_bDChrgCoolAbnorm/1 -> MaxCurrCalc/5(BCMR_bDChrgCoolAbnorm), [BCMR_bDChrgCoolAbnorm]
  [BCMR_bDChrgCoolAbnorm] -> MixCurrCalc2/5(BCMR_bDChrgCoolAbnorm)
  BSER_rSoh/1 -> [BSER_rSoh], MaxCurrCalc/1(BSER_rSoh)
  [BSER_rSoh] -> MixCurrCalc2/1(BSER_rSoh)
  [BCMR_uDcChrgCellVolt_A] -> MixCurrCalc2/4(BCMR_uDcChrgCellVolt_A)
  BCMR_tDcChrgCellTemp_A/1 -> [BCMR_tDcChrgCellTemp_A], MaxCurrCalc/6(BCMR_tDcChrgCellTemp_A)
  BCMR_bDChrgDistLmt/1 -> [BCMR_bDChrgDistLmt], MaxCurrCalc/7(BCMR_bDChrgDistLmt)
  [BCMR_tDcChrgCellTemp_A] -> MixCurrCalc2/6(BCMR_tDcChrgCellTemp_A)
  [BCMR_bDChrgDistLmt] -> MixCurrCalc2/7(BCMR_bDChrgDistLmt)
  [BCMR_flgDChrgFulChk] -> MaxCurrCalc/8(BCMR_flgDChrgFulChk)
  [BCMR_flgDChrgFulChk] -> MixCurrCalc2/8(BCMR_flgDChrgFulChk)
  COMR_iDcChrgOutputCurrCcs/1 -> CurrCalc/8(COMR_iDcChrgOutputCurrCcs)
  COMR_iDcChrgMinCurrOutputPmtdCml/1 -> CurrCalc/9(COMR_iDcChrgMinCurrOutputPmtdCml)
  [BSPR_uCellVoltMax] -> CurrSpTemp/2(BSPR_uCellVoltMax)
  [BCMR_bDChrgDistLmt] -> CurrSpTemp/3(BCMR_bDChrgDistLmt)
  [BCMR_bDChrgCoolAbnorm] -> CurrSpTemp/4(BCMR_bDChrgCoolAbnorm)
  CurrMerge/1(Out1) -> Switch/1
  Switch/1 -> CurrCalc/1(Curr)
  CurrSpTemp/1(BCMR_iBattDCCurrReqFinal) -> Switch/3
  Constant1/1 -> Switch/2
  BCMR_bDChrgCurrReqEna/1 -> CurrSpTemp/5(BCMR_bDChrgCurrReqEna)
  BCMR_bDChrgStopEna/1 -> CurrSpTemp/6(BCMR_bDChrgStopEna)
  BCMR_stDChrgMode/1 -> CurrCalc/10(BCMR_stDChrgMode)
  Mux/1 -> CurrSpTemp/1(BSPR_tBattTemp)
  [BSPR_tBattTempMax] -> Mux/1
  [BSPR_tBattTempMin] -> Mux/2
  BSPR_iBattCurr/1 -> CurrSpTemp/7(BSPR_iBattCurr)

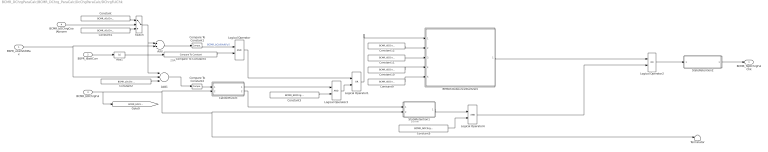
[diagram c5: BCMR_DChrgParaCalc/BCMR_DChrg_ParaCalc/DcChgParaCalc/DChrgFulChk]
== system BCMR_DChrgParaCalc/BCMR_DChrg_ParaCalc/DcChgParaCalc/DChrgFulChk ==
  note: 20A
  note: 10min
  BSPR_uCellVoltMax : Inport
  BSPR_iBattCurr : Inport  Port=2
  BCMR_bDChrgFul : Inport  Port=3
  BCMR_bDChrgCoolAbnorm : Inport  Port=4
  Abs1 : Abs
  Add : Sum  Inputs=-+
  Add1 : Sum  Inputs=-+-
  BMSDCDebounceStartZero : Subsystem  AncestorBlock=AIWAYS_Powertrain_BMS_lib/Debounce & Delay/BMSDebounceStartZero  TreatAsAtomicUnit=on
  CellVoltFulCnt : Subsystem  TreatAsAtomicUnit=on
  Compare To Constant1 : simulink/Logic and Bit Operations/Compare To Constant  relop=>=  const=0  OutDataTypeStr=boolean
  Compare To Constant2 : simulink/Logic and Bit Operations/Compare To Constant  relop=>=  const=0  OutDataTypeStr=boolean
  Compare To Constant4 : simulink/Logic and Bit Operations/Compare To Constant  relop=<  const=BCMR_iDChrgCurrCutOff_C  OutDataTypeStr=boolean
  Constant : Constant  Value=BCMR_vDcChrgFullCellVoltCool_C
  Constant1 : Constant  Value=BCMR_vDcChrgFullCellVolt_C
  Constant10 : Constant  Value=BCMR_tiDChrgFullDebs_C
  Constant11 : Constant  Value=BCMR_tiDChrgFullBase_C
  Constant12 : Constant  Value=BCMR_tiDChrgFullDebs_C
  Constant2 : Constant  Value=BCMR_uDcChrgFullCellVoltOff_C
  Constant3 : Constant  Value=BCMR_bDChrgFulChkTenEna_C
  Constant5 : Constant  Value=BCMR_bDChrgFulChkThreeEna_C
  Constant9 : Constant  Value=BCMR_tiDChrgFullBase_C
  Logical Operator : Logic  AllPortsSameDT=off  OutDataTypeStr=boolean
  Logical Operator1 : Logic  Operator=OR  AllPortsSameDT=off  OutDataTypeStr=boolean
  Logical Operator2 : Logic  Operator=OR  AllPortsSameDT=off  OutDataTypeStr=boolean
  Logical Operator3 : Logic  AllPortsSameDT=off  OutDataTypeStr=boolean
  Logical Operator4 : Logic  AllPortsSameDT=off  OutDataTypeStr=boolean
  StateRetention1 : Subsystem
  StateRetention2 : Subsystem
  Switch : Switch  Criteria=u2 > Threshold
  Terminator : Terminator
  BCMR_flgDChrgFulChk : Outport
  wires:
  BSPR_iBattCurr/1 -> Abs1/1
  Abs1/1 -> Compare To Constant4/1
  Compare To Constant4/1 -> Logical Operator/2
  StateRetention2/1(BCMR_flgDChrgFulChk) -> BCMR_flgDChrgFulChk/1
  Logical Operator/1 -> Logical Operator1/1
  Compare To Constant1/1 -> Logical Operator/1  "BCMR_bCellVoltFull"
  Constant/1 -> Switch/1
  BCMR_bDChrgCoolAbnorm/1 -> Switch/2
  Constant1/1 -> Switch/3
  Add/1 -> Compare To Constant1/1
  Switch/1 -> Add1/1, Add/1
  BSPR_uCellVoltMax/1 -> Add1/2, Add/2
  CellVoltFulCnt/1(Ten) -> Logical Operator3/1
  BCMR_bDChrgFul/1 -> Terminator/1, StateRetention1/2(clc), CellVoltFulCnt/2(Rst), [BCMR_bDChrgFul]
  StateRetention1/1(BCMR_bCellVoltFullTmr) -> Logical Operator4/1
  Logical Operator2/1 -> StateRetention2/1(u)
  CellVoltFulCnt/2(Three) -> StateRetention1/1(u)
  Add1/1 -> Compare To Constant2/1
  Compare To Constant2/1 -> CellVoltFulCnt/1(En)
  Constant2/1 -> Add1/3
  Logical Operator3/1 -> Logical Operator1/2
  Constant3/1 -> Logical Operator3/2
  Constant5/1 -> Logical Operator4/2
  Logical Operator1/1 -> BMSDCDebounceStartZero/1(Signal)
  Constant11/1 -> BMSDCDebounceStartZero/3(FaultStep)
  Constant12/1 -> BMSDCDebounceStartZero/2(Hearl2Fault)
  Constant9/1 -> BMSDCDebounceStartZero/5(HealStep)
  Constant10/1 -> BMSDCDebounceStartZero/4(Fault2Heal)
  Logical Operator4/1 -> Logical Operator2/2
  BMSDCDebounceStartZero/1(FaultFlag) -> Logical Operator2/1

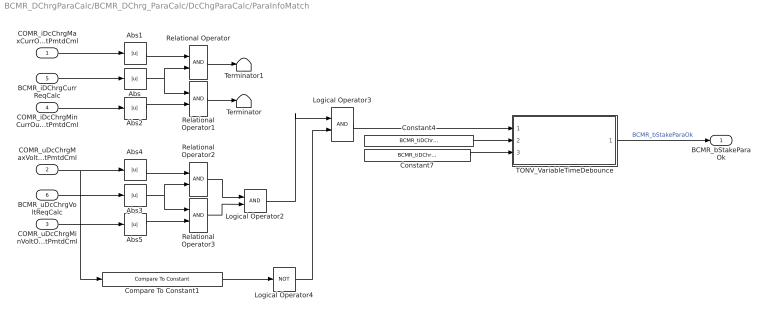
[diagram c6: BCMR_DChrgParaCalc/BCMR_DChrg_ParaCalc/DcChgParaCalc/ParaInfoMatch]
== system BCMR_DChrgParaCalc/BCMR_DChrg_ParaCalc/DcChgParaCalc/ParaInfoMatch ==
  COMR_iDcChrgMaxCurrOutputPmtdCml : Inport
  COMR_uDcChrgMaxVoltOutputPmtdCml : Inport  Port=2
  COMR_uDcChrgMinVoltOutputPmtdCml : Inport  Port=3
  COMR_iDcChrgMinCurrOutputPmtdCml : Inport  Port=4
  BCMR_iDChrgCurrReqCalc : Inport  Port=5
  BCMR_uDcChrgVoltReqCalc : Inport  Port=6
  Abs{,1..5} (6 alike) : Abs
  Compare To Constant1 : simulink/Logic and Bit Operations/Compare To Constant  relop=<=  const=BMCR_uDChrgerVoltMish_C  OutDataTypeStr=boolean
  Constant4 : Constant  Value=BCMR_tiDChrgDetParaDebs_C
  Constant7 : Constant  Value=BCMR_tiDChrgParaBase_C
  Logical Operator2 : Logic  AllPortsSameDT=off  OutDataTypeStr=boolean
  Logical Operator3 : Logic  AllPortsSameDT=off  OutDataTypeStr=boolean
  Logical Operator4 : Logic  Operator=NOT  AllPortsSameDT=off  OutDataTypeStr=boolean
  Relational Operator{,1..3} (4 alike) : RelationalOperator  OutDataTypeStr=boolean  RndMeth=Simplest
  TONV_VariableTimeDebounce : Subsystem  TreatAsAtomicUnit=on  RTWFcnName=TONV_VariableTimeDebounce  RTWFileName=SrvLib
  Terminator : Terminator
  Terminator1 : Terminator
  BCMR_bStakeParaOk : Outport
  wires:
  Logical Operator2/1 -> Logical Operator3/1
  Abs5/1 -> Relational Operator3/2
  Abs1/1 -> Relational Operator/1
  Abs3/1 -> Relational Operator2/2, Relational Operator3/1
  COMR_iDcChrgMaxCurrOutputPmtdCml/1 -> Abs1/1
  Abs2/1 -> Relational Operator1/2
  COMR_uDcChrgMinVoltOutputPmtdCml/1 -> Abs5/1
  Abs/1 -> Relational Operator1/1, Relational Operator/2
  Relational Operator3/1 -> Logical Operator2/2
  COMR_iDcChrgMinCurrOutputPmtdCml/1 -> Abs2/1
  TONV_VariableTimeDebounce/1(y) -> BCMR_bStakeParaOk/1  "BCMR_bStakeParaOk"
  COMR_uDcChrgMaxVoltOutputPmtdCml/1 -> Compare To Constant1/1, Abs4/1
  BCMR_iDChrgCurrReqCalc/1 -> Abs/1
  Relational Operator2/1 -> Logical Operator2/1
  BCMR_uDcChrgVoltReqCalc/1 -> Abs3/1
  Abs4/1 -> Relational Operator2/1
  Logical Operator3/1 -> TONV_VariableTimeDebounce/1(u)
  Constant7/1 -> TONV_VariableTimeDebounce/3(dT)
  Compare To Constant1/1 -> Logical Operator4/1
  Logical Operator4/1 -> Logical Operator3/2
  Relational Operator1/1 -> Terminator/1
  Constant4/1 -> TONV_VariableTimeDebounce/2(T)
  Relational Operator/1 -> Terminator1/1

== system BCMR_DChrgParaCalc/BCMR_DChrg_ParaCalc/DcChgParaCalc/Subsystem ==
  COMR_stVcuFalutLvl : Inport
  DSMR_stFaultRank : Inport  Port=2
  Compare To Constant1 : simulink/Logic and Bit Operations/Compare To Constant  relop===  const=2  OutDataTypeStr=boolean
  Compare To Constant2 : simulink/Logic and Bit Operations/Compare To Constant  relop===  const=2  OutDataTypeStr=boolean
  Constant4 : Constant  Value=BCMR_tiDChrgDetParaDebs_C
  Constant7 : Constant  Value=BCMR_tiDChrgParaBase_C
  Logical Operator1 : Logic  Operator=OR  AllPortsSameDT=off  OutDataTypeStr=boolean
  TONV_VariableTimeDebounce1 : Subsystem  TreatAsAtomicUnit=on  RTWFcnName=TONV_VariableTimeDebounce  RTWFileName=SrvLib
  BCMR_flgDChrgPwrRdc : Outport
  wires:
  Compare To Constant1/1 -> Logical Operator1/1
  TONV_VariableTimeDebounce1/1(y) -> BCMR_flgDChrgPwrRdc/1  "BCMR_flgDChrgPwrRdc"
  COMR_stVcuFalutLvl/1 -> Compare To Constant1/1
  Compare To Constant2/1 -> Logical Operator1/2
  DSMR_stFaultRank/1 -> Compare To Constant2/1
  Logical Operator1/1 -> TONV_VariableTimeDebounce1/1(u)
  Constant4/1 -> TONV_VariableTimeDebounce1/2(T)
  Constant7/1 -> TONV_VariableTimeDebounce1/3(dT)

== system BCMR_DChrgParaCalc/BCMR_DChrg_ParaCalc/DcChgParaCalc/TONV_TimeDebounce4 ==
  note: Turn On Delay Time Deboune
  T : Inport
  u : Inport  Port=2
  dT : Inport  Port=3
  Add : Sum
  Constant1 : Constant  Value=0  OutDataTypeStr=uint8
  Constant2 : Constant  OutDataTypeStr=uint8
  Constant3 : Constant  Value=0  OutDataTypeStr=single
  Delay : Delay  DelayLength=1  InitialCondition=0
  MinMax : MinMax  Inputs=2
  Product : Product  OutMin=[0]  OutMax=[65535]  OutDataTypeStr=single
  Relational Operator : RelationalOperator  OutDataTypeStr=boolean  RndMeth=Simplest
  Switch : Switch  Criteria=u2 ~= 0
  Switch1 : Switch  Criteria=u2 ~= 0
  y : Outport
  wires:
  u/1 -> Switch1/2, Switch/2
  Switch/1 -> Product/1
  dT/1 -> Switch1/1
  Constant3/1 -> Switch1/3
  Constant2/1 -> Switch/1
  Constant1/1 -> Switch/3
  Add/1 -> Product/2
  Product/1 -> Relational Operator/1, Delay/1
  Switch1/1 -> Add/1
  Delay/1 -> MinMax/2
  Relational Operator/1 -> y/1
  T/1 -> Relational Operator/2, MinMax/1
  MinMax/1 -> Add/2

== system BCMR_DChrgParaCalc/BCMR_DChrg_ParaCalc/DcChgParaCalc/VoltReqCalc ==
  COMR_uDcChrgMaxVoltOutputPmtdCml : Inport
  COMR_uDcChrgMinVoltOutputPmtdCml : Inport  Port=2
  BSPR_uBattVolt : Inport  Port=3
  Add : Sum
  Constant1 : Constant  Value=BCMR_uBattVoltOff_C
  Constant2 : Constant  Value=BCMR_uDChrgVoltReq_C  OutDataTypeStr=single
  MinMax : MinMax  Inputs=3
  MinMax1 : MinMax  Function=max  Inputs=2
  BCMR_uDcChrgVoltReqCalc : Outport
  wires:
  COMR_uDcChrgMinVoltOutputPmtdCml/1 -> MinMax1/2
  Constant2/1 -> MinMax/2
  COMR_uDcChrgMaxVoltOutputPmtdCml/1 -> MinMax1/1
  MinMax1/1 -> MinMax/1
  BSPR_uBattVolt/1 -> Add/1
  Constant1/1 -> Add/2
  Add/1 -> MinMax/3
  MinMax/1 -> BCMR_uDcChrgVoltReqCalc/1

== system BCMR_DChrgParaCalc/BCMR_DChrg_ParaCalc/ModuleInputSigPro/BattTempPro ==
  BSPR_tBattTempMin : Inport
  BSPR_tBattTempMax : Inport  Port=2
  Compare To Constant2 : simulink/Logic and Bit Operations/Compare To Constant  relop=<  const=BCMR_tBattTempSelcLmtDwn_C  OutDataTypeStr=boolean
  Compare To Constant3 : simulink/Logic and Bit Operations/Compare To Constant  relop=<  const=BCMR_tBattTempSelcLmtDwn_C  OutDataTypeStr=boolean
  Compare To Constant4 : simulink/Logic and Bit Operations/Compare To Constant  relop=>=  const=BCMR_tBattTempSelcLmtUp_C  OutDataTypeStr=boolean
  Constant1 : Constant  Value=BCMR_uDcChrgCellVolt1_A  OutDataTypeStr=single
  Constant2 : Constant  Value=BCMR_uDcChrgCellVolt3_A  OutDataTypeStr=single
  Constant3 : Constant  Value=BCMR_uDcChrgCellVolt2_A  OutDataTypeStr=single
  Constant4 : Constant  Value=BCMR_tiDChrgParaBase_C
  Constant5 : Constant  Value=BCMR_tiBattTempSwitch_C
  Constant6 : Constant  Value=BCMR_tiBattTempSwitch_C
  Constant7 : Constant  Value=BCMR_tiDChrgParaBase_C
  Switch1 : Switch  Criteria=u2 > Threshold
  Switch3 : Switch  Criteria=u2 > Threshold
  Switch5 : Switch  Criteria=u2 > Threshold
  TONV_VariableTimeDebounce : Subsystem  TreatAsAtomicUnit=on  RTWFcnName=TONV_VariableTimeDebounce  RTWFileName=SrvLib
  TONV_VariableTimeDebounce1 : Subsystem  TreatAsAtomicUnit=on  RTWFcnName=TONV_VariableTimeDebounce  RTWFileName=SrvLib
  BCMR_uDcChrgCellVolt_A : Outport
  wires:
  BSPR_tBattTempMin/1 -> Switch5/1, Compare To Constant3/1
  Compare To Constant3/1 -> Switch5/2
  BSPR_tBattTempMax/1 -> Switch5/3
  Constant1/1 -> Switch1/1
  Constant2/1 -> Switch3/1
  Constant3/1 -> Switch3/3
  Switch3/1 -> Switch1/3
  Switch1/1 -> BCMR_uDcChrgCellVolt_A/1
  TONV_VariableTimeDebounce/1(y) -> Switch1/2
  Compare To Constant2/1 -> TONV_VariableTimeDebounce/1(u)
  Compare To Constant4/1 -> TONV_VariableTimeDebounce1/1(u)
  TONV_VariableTimeDebounce1/1(y) -> Switch3/2
  Constant7/1 -> TONV_VariableTimeDebounce/3(dT)
  Constant4/1 -> TONV_VariableTimeDebounce1/3(dT)
  Constant5/1 -> TONV_VariableTimeDebounce/2(T)
  Constant6/1 -> TONV_VariableTimeDebounce1/2(T)
  Switch5/1 -> Compare To Constant2/1, Compare To Constant4/1

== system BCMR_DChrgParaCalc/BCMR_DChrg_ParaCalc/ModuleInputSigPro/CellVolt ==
  BSPR_uCellVoltMax : Inport
  BSPR_uCellVoltMin : Inport  Port=2
  Compare To Constant1 : simulink/Logic and Bit Operations/Compare To Constant  relop=<  const=BCMR_uCellVoltHiValVld_C  OutDataTypeStr=boolean
  Compare To Constant2 : simulink/Logic and Bit Operations/Compare To Constant  relop=<  const=BCMR_uCellVoltHiValVld_C  OutDataTypeStr=boolean
  Compare To Constant3 : simulink/Logic and Bit Operations/Compare To Constant  relop=>  const=BCMR_uCellVoltLoValVld_C  OutDataTypeStr=boolean
  Compare To Constant4 : simulink/Logic and Bit Operations/Compare To Constant  relop=>  const=BCMR_uCellVoltLoValVld_C  OutDataTypeStr=boolean
  Logical Operator : Logic  AllPortsSameDT=off  OutDataTypeStr=boolean
  Logical Operator1 : Logic  AllPortsSameDT=off  OutDataTypeStr=boolean
  Switch : Switch  Criteria=u2 ~= 0
  Switch1 : Switch  Criteria=u2 ~= 0
  Unit Delay : UnitDelay  SampleTime=-1
  Unit Delay1 : UnitDelay  SampleTime=-1
  BCMR_uCellVoltMin : Outport
  BCMR_uCellVoltMax : Outport  Port=2
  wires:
  Switch/1 -> Unit Delay/1, BCMR_uCellVoltMin/1
  BSPR_uCellVoltMin/1 -> Compare To Constant4/1, Compare To Constant2/1, Switch/1
  Compare To Constant2/1 -> Logical Operator/1
  Compare To Constant4/1 -> Logical Operator/2
  Logical Operator/1 -> Switch/2
  Unit Delay/1 -> Switch/3
  Switch1/1 -> BCMR_uCellVoltMax/1, Unit Delay1/1
  BSPR_uCellVoltMax/1 -> Switch1/1, Compare To Constant1/1, Compare To Constant3/1
  Compare To Constant1/1 -> Logical Operator1/1
  Compare To Constant3/1 -> Logical Operator1/2
  Logical Operator1/1 -> Switch1/2
  Unit Delay1/1 -> Switch1/3

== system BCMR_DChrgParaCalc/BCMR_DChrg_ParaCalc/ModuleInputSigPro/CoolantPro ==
  DFC_CoolPerfPlaus : Inport
  Bitwise Operator6 : simulink/Logic and Bit Operations/Bitwise Operator  logicop=AND  UseBitMask=on  BitMask=bin2dec('00011000')  BitMaskRealWorld=Stored Integer
  Compare To Constant2 : simulink/Logic and Bit Operations/Compare To Constant  relop===  const=24  OutDataTypeStr=boolean
  Constant : Constant  Value=BCMR_cntCoolDFC_CW
  Constant1 : Constant  OutDataTypeStr=boolean
  Constant2 : Constant  Value=BCMR_tDcChrgCellTemp2_A
  Constant3 : Constant  Value=BCMR_tDcChrgCellTemp1_A
  Switch : Switch  Criteria=u2 > Threshold  Threshold=6
  Switch1 : Switch  Criteria=u2 > Threshold  Threshold=6
  BCMR_bDChrgCoolAbnorm : Outport
  BCMR_uDcChrgCellTemp_A : Outport  Port=2
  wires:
  Bitwise Operator6/1 -> Compare To Constant2/1
  Constant1/1 -> Switch/3
  Switch/1 -> Switch1/2, BCMR_bDChrgCoolAbnorm/1
  Constant/1 -> Switch/2
  DFC_CoolPerfPlaus/1 -> Bitwise Operator6/1
  Compare To Constant2/1 -> Switch/1
  Constant2/1 -> Switch1/1
  Constant3/1 -> Switch1/3
  Switch1/1 -> BCMR_uDcChrgCellTemp_A/1

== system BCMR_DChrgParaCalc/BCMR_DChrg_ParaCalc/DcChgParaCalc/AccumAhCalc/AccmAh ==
  BSPR_iBattCurr : Inport
  Abs1 : Abs
  Add4 : Sum
  Data Type Conversion : DataTypeConversion  OutDataTypeStr=single
  Gain : Gain  Gain=1/360000
  IC : InitialCondition  Value=0
  Unit Delay4 : UnitDelay  SampleTime=-1
  BCMR_ahDChrgAhAccum : Outport
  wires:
  BSPR_iBattCurr/1 -> Abs1/1
  Abs1/1 -> Add4/2
  Unit Delay4/1 -> Add4/1
  Data Type Conversion/1 -> BCMR_ahDChrgAhAccum/1
  IC/1 -> Data Type Conversion/1
  Gain/1 -> IC/1
  Add4/1 -> Gain/1, Unit Delay4/1

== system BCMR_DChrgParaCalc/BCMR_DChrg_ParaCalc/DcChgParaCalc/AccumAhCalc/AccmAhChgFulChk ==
  BCMR_rSocInit : Inport
  BCMR_ahAccumDChrgAh : Inport  Port=2
  Add : Sum
  Constant4 : Constant  Value=BCMR_ahDChgBattNominalCapa_C
  Gain : Gain  Gain=0.01
  Gain1 : Gain  Gain=BCMR_ahDChgBattNominalCapa_C
  Gain2 : Gain  Gain=0.9
  Relational Operator : RelationalOperator  OutDataTypeStr=boolean  RndMeth=Simplest
  BCMR_bAccumAhDChrgFul : Outport
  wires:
  Relational Operator/1 -> BCMR_bAccumAhDChrgFul/1  "BCMR_bAccumAhDChrgFul"
  Add/1 -> Relational Operator/1
  BCMR_ahAccumDChrgAh/1 -> Add/2
  BCMR_rSocInit/1 -> Gain/1
  Gain/1 -> Gain1/1
  Gain1/1 -> Add/1
  Constant4/1 -> Gain2/1
  Gain2/1 -> Relational Operator/2

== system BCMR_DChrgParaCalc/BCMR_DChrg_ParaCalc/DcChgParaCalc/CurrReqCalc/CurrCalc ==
  Curr : Inport
  COMR_iDcChrgMaxCurrOutputPmtdCml : Inport  Port=2
  BCMR_flgDChrgPwrRdc : Inport  Port=3
  COMR_tiDcChrgTimeActualCcs : Inport  Port=4
  COMR_pwrChrgLdReq : Inport  Port=5
  BSPR_uPackVolt : Inport  Port=6
  BSPR_tBattTempMin : Inport  Port=7
  COMR_iDcChrgOutputCurrCcs : Inport  Port=8
  COMR_iDcChrgMinCurrOutputPmtdCml : Inport  Port=9
  BCMR_stDChrgMode : Inport  Port=10
  Add : Sum
  BattCurrReq : Subsystem
  BattCurrReq1 : Subsystem
  LoadCurrReq : Subsystem
  BCMR_iDChrgBattCurrReqCalc : Outport
  BCMR_iDChrgLoadCurrReqCalc : Outport  Port=2
  BCMR_iDChrgCurrReqCalc : Outport  Port=3
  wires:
  Curr/1 -> BattCurrReq/1(Curr)
  BCMR_flgDChrgPwrRdc/1 -> BattCurrReq/2(BCMR_flgDChrgPwrRdc)
  BattCurrReq/1(BCMR_iDChrgBattCurrReqCalc) -> Add/1, BCMR_iDChrgBattCurrReqCalc/1
  COMR_pwrChrgLdReq/1 -> LoadCurrReq/1(COMR_pwrChrgLdReq)
  BSPR_uPackVolt/1 -> [BSPR_uPackVolt], LoadCurrReq/2(BSPR_uPackVolt)
  BSPR_tBattTempMin/1 -> LoadCurrReq/3(BSPR_tBattTempMin)
  LoadCurrReq/1(BCMR_iDChrgLoadCurrReqCalc) -> Add/2, BCMR_iDChrgLoadCurrReqCalc/1
  BattCurrReq1/1(BCMR_iDChrgBattCurrReqCalc) -> BCMR_iDChrgCurrReqCalc/1
  Add/1 -> BattCurrReq1/1(CurrReq)
  [BSPR_uPackVolt] -> BattCurrReq1/6(BSPR_uPackVolt)
  COMR_iDcChrgMaxCurrOutputPmtdCml/1 -> BattCurrReq1/2(COMR_iDcChrgMaxCurrOutputPmtdCml)
  COMR_tiDcChrgTimeActualCcs/1 -> BattCurrReq1/3(COMR_tiDcChrgTimeActualCcs)
  COMR_iDcChrgOutputCurrCcs/1 -> BattCurrReq1/4(COMR_iDcChrgOutputCurrCcs)
  COMR_iDcChrgMinCurrOutputPmtdCml/1 -> BattCurrReq1/5(COMR_iDcChrgMinCurrOutputPmtdCml)
  BCMR_stDChrgMode/1 -> BattCurrReq1/7(BCMR_stDChrgMode)

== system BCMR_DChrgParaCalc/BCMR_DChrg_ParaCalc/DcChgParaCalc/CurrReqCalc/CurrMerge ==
  In1 : Inport
  In2 : Inport  Port=2
  ShadeFall : Subsystem
  Out1 : Outport
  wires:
  ShadeFall/1(val) -> Out1/1
  In2/1 -> ShadeFall/2(In2)
  In1/1 -> ShadeFall/1(In1)

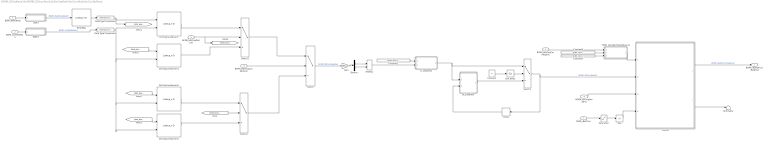
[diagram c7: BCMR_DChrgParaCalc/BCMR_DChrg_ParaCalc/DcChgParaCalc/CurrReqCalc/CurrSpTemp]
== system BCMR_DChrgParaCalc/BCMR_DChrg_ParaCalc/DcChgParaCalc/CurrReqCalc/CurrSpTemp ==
  BSPR_tBattTemp : Inport
  BSPR_uCellVoltMax : Inport  Port=2
  BCMR_bDChrgDistLmt : Inport  Port=3
  BCMR_bDChrgCoolAbnorm : Inport  Port=4
  BCMR_bDChrgCurrReqEna : Inport  Port=5
  BCMR_bDChrgStopEna : Inport  Port=6
  BSPR_iBattCurr : Inport  Port=7
  Abs : Abs
  Constant : Constant  Value=0  OutDataTypeStr=boolean
  Constant2 : Constant  Value=BCMR_iDCCurrFil_C  OutDataTypeStr=single
  Constant5 : Constant  Value=BCMR_tiDChrgCurrReqCalDly_C
  Constant7 : Constant  Value=BCMR_tiDChrgParaBase_C
  CurrFilt : Stateflow chart  TreatAsAtomicUnit=on
  "DCChrgFilter " : Subsystem
  Data Type Conversion : DataTypeConversion  OutDataTypeStr=single
  Data Type Conversion1 : DataTypeConversion  OutDataTypeStr=single
  DcChrgCurrAbnorm : Lookup_n-D  BreakpointsForDimension1=BCMR_tDcChrgCellTemp_A  BreakpointsForDimension2=BCMR_uDcChrgCellVoltOld_A  Table=BCMR_iDcChrgCurrOldAbnormMAP_T  ExtrapMethod=Clip  UseLastTableValue=on  InternalRulePriority=Speed  RndMeth=Simplest
  DcChrgCurrAbnorm1 : Lookup_n-D  BreakpointsForDimension1=BCMR_tDcChrgCellTemp_A  BreakpointsForDimension2=BCMR_uDcChrgCellVoltNew_A  Table=BCMR_iDcChrgCurrAbnormMAP_T  ExtrapMethod=Clip  UseLastTableValue=on  InternalRulePriority=Speed  RndMeth=Simplest
  DcChrgCurrAbnorm2 : Lookup_n-D  BreakpointsForDimension1=BCMR_tDcChrgCellTemp_A  BreakpointsForDimension2=BCMR_uDcChrgCellVoltOld_A  Table=BCMR_iDcChrgCurrOldMAP_T  ExtrapMethod=Clip  UseLastTableValue=on  InternalRulePriority=Speed  RndMeth=Simplest
  DcChrgCurrAbnorm3 : Lookup_n-D  BreakpointsForDimension1=BCMR_tDcChrgCellTemp_A  BreakpointsForDimension2=BCMR_uDcChrgCellVoltNew_A  Table=BCMR_iDcChrgCurrNewMAP_T  ExtrapMethod=Clip  UseLastTableValue=on  InternalRulePriority=Speed  RndMeth=Simplest
  Delay : Delay  DelayLength=1  InitialCondition=0
  Demux : Demux  Outputs=2
  Gain : Gain  Gain=BCMR_ahDChgBattNominalCapa_C
  K_Lowpass2 : Subsystem  TreatAsAtomicUnit=on  RTWFcnName=K_Lowpass  RTWFileName=SrvLib
  MinMax : MinMax  Inputs=2
  SIgFil : Subsystem
  SIgFil1 : Subsystem
  Saturation : Saturate  UpperLimit=0  LowerLimit=-inf
  Switch{,1..3} (4 alike) : Switch  Criteria=u2 ~= 0
  TONV_VariableTimeDebounce : Subsystem  TreatAsAtomicUnit=on  RTWFcnName=TONV_VariableTimeDebounce  RTWFileName=SrvLib
  TempMap : Lookup_n-D  NumberOfTableDimensions=1  BreakpointsForDimension1=BCMR_tTempDisMapX_A  BreakpointsForDimension2=BCMR_uDcChrgCellVolt1_A  Table=BCMR_tTempDisMapY_A  InterpMethod=Flat  ExtrapMethod=Clip  UseLastTableValue=on  InternalRulePriority=Speed  RndMeth=Simplest
  Terminator : Terminator
  Unit Delay : UnitDelay  InitialCondition=1  SampleTime=-1
  BCMR_iBattDCCurrReqFinal : Outport
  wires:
  SIgFil/1(y) -> TempMap/1  "BCMR_tBattTempMaxFil"
  [BSPR_tBattTempMax] -> DcChrgCurrAbnorm1/1
  SIgFil1/1(y) -> Data Type Conversion1/1  "BCMR_uCellVoltMaxFil"
  BCMR_bDChrgCoolAbnorm/1 -> Switch/2
  Switch1/1 -> Switch/1
  Switch2/1 -> Switch/3
  BCMR_bDChrgDistLmt/1 -> [BCMR_bDChrgDistLmt], Switch1/2
  DcChrgCurrAbnorm/1 -> Switch1/1
  DcChrgCurrAbnorm1/1 -> Switch1/3
  DcChrgCurrAbnorm2/1 -> Switch2/1
  DcChrgCurrAbnorm3/1 -> Switch2/3
  [BSPR_tBattTempMax] -> DcChrgCurrAbnorm2/1
  [BSPR_tBattTempMax] -> DcChrgCurrAbnorm3/1
  [BCMR_bDChrgDistLmt] -> Switch2/2
  Switch3/1 -> CurrFilt/2(DCCurrReqIn), Delay/1  "BCMR_iDCCurrReqFil2"
  Delay/1 -> "DCChrgFilter "/2(In2)
  "DCChrgFilter "/1(Out1) -> Switch3/3
  Switch/1 -> Gain/1  "BCMR_iDCCurrReqRaw"
  CurrFilt/1(DCCurrReq) -> BCMR_iBattDCCurrReqFinal/1  "BCMR_iBattDCCurrReqFinal"
  CurrFilt/2(DCCurrTarget) -> Terminator/1
  Unit Delay/1 -> Switch3/2
  Constant/1 -> Unit Delay/1
  BCMR_bDChrgStopEna/1 -> CurrFilt/3(DCChrgStop)
  Constant7/1 -> TONV_VariableTimeDebounce/3(dT)
  Constant5/1 -> TONV_VariableTimeDebounce/2(T)
  BCMR_bDChrgCurrReqEna/1 -> TONV_VariableTimeDebounce/1(u)
  TONV_VariableTimeDebounce/1(y) -> CurrFilt/1(DCChrgEn)
  Constant2/1 -> K_Lowpass2/1(k)
  BSPR_tBattTemp/1 -> SIgFil/1(u)
  BSPR_uCellVoltMax/1 -> SIgFil1/1(u)
  Data Type Conversion/1 -> [BSPR_tBattTempMax], DcChrgCurrAbnorm/1
  Data Type Conversion1/1 -> DcChrgCurrAbnorm2/2, DcChrgCurrAbnorm3/2, DcChrgCurrAbnorm1/2, DcChrgCurrAbnorm/2
  TempMap/1 -> Data Type Conversion/1
  Gain/1 -> Demux/1
  Demux/1 -> MinMax/1
  Demux/2 -> MinMax/2
  K_Lowpass2/1(y) -> "DCChrgFilter "/1(In1), Switch3/1
  MinMax/1 -> K_Lowpass2/2(u)
  BSPR_iBattCurr/1 -> Saturation/1
  Saturation/1 -> Abs/1
  Abs/1 -> CurrFilt/4(BSPR_iBattCurr)
